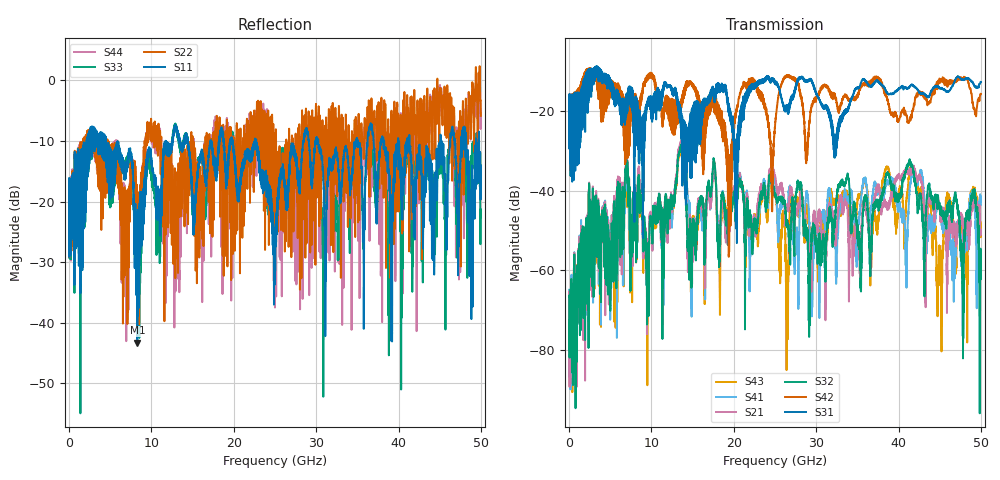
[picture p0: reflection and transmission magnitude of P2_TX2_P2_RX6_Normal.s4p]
!Keysight Technologies,N5225B,MY57041031,A.13.20.10
!Date: Friday, May 31, 2019 11:35:54
!Correction: S11(Full 4 Port(1,2,3,4))
!S12(Full 4 Port(1,2,3,4))
!S13(Full 4 Port(1,2,3,4))
!S14(Full 4 Port(1,2,3,4))
!S21(Full 4 Port(1,2,3,4))
!S22(Full 4 Port(1,2,3,4))
!S23(Full 4 Port(1,2,3,4))
!S24(Full 4 Port(1,2,3,4))
!S31(Full 4 Port(1,2,3,4))
!S32(Full 4 Port(1,2,3,4))
!S33(Full 4 Port(1,2,3,4))
!S34(Full 4 Port(1,2,3,4))
!S41(Full 4 Port(1,2,3,4))
!S42(Full 4 Port(1,2,3,4))
!S43(Full 4 Port(1,2,3,4))
!S44(Full 4 Port(1,2,3,4))
!S4P File: Measurements: <S11,S12,S13,S14>,
!<S21,S22,S23,S24>,
!<S31,S32,S33,S34>,
!<S41,S42,S43,S44>:
# Hz S  dB  R 50.0
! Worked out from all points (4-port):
!   5000 points, 10 MHz to 50 GHz, reference 50 ohm
!   strongest paths, dB at 10 MHz, 12.51 GHz, 25.01 GHz, 37.51 GHz, 50 GHz:
!     S31: -19.4, -14.8, -13.0, -12.4, -12.6
!     S42: -19.5, -16.9, -23.7, -11.3, -15.6
!     S32: -66.7, -44.6, -41.2, -42.6, -55.5
!     S21: -71.6, -43.7, -36.1, -38.6, -50.5
!     S41: -64.9, -46.7, -37.7, -39.8, -43.6
!     S43: -82.9, -47.6, -41.0, -46.9, -49.3
!   lowest |S11| = -43.3 dB at 8.29 GHz (marker M1), VSWR 1.01, Z = 49.9 + j0.679 ohm
!   |S11| at or under -10 dB: 4.481 GHz to 11.72 GHz (7.237 GHz wide, 89.4 % of centre); 22.73 GHz to 28.43 GHz (5.703 GHz wide, 22.3 % of centre); 30.26 GHz to 34.82 GHz (4.56 GHz wide, 14 % of centre)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
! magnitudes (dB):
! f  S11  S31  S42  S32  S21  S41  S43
! 10 MHz  -19.2  -19.4  -19.5  -66.7  -71.6  -64.9  -82.9
! 8.29 GHz  -43.3  -18.8  -19.2  -43.3  -42.3  -42.8  -44.0
! 27.97 GHz  -16.7  -11.6  -14.5  -38.8  -43.2  -48.9  -44.6
! 29.23 GHz  -12.2  -12.1  -22.2  -61.0  -54.0  -51.5  -52.0
! 41.42 GHz  -11.0  -13.6  -22.1  -32.8  -35.7  -38.0  -34.2
! 44.97 GHz  -10.3  -14.0  -11.7  -43.7  -44.5  -43.9  -53.8
! 50 GHz  -14.0  -12.6  -15.6  -55.5  -50.5  -43.6  -49.3
